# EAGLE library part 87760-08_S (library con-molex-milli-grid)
HEADER
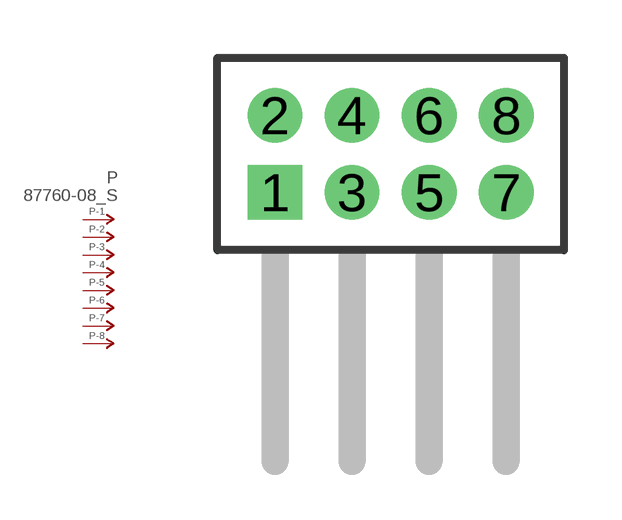
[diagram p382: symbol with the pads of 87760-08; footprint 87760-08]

Designator prefix P; gates -1=P-NV -2=P-N -3=P-N -4=P-N -5=P-N -6=P-N -7=P-N -8=P-N

## 87760-08_S  [87760-08]
1  -1:P  pas
2  -2:P  pas
3  -3:P  pas
4  -4:P  pas
5  -5:P  pas
6  -6:P  pas
7  -7:P  pas
8  -8:P  pas

## Footprint 87760-08 (pad centres in mm)
HEADER Dual Row, Right Angle
drill 0.914 square: 1 -3,-1
drill 0.914: 2 -3,1; 3 -1,-1; 4 -1,1; 5 1,-1; 6 1,1; 7 3,-1; 8 3,1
